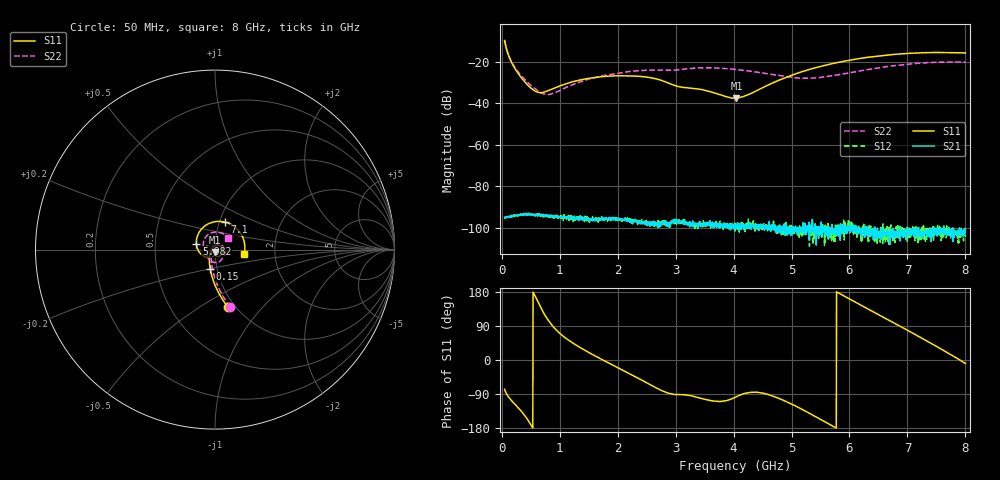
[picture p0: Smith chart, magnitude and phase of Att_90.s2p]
#  HZ  S  DB  R  50.00
! Rohde & Schwarz Vector Network Analyzer
! Rohde-Schwarz,ZNB40-4Port,1311601084101679,3.45
! Created: UTC 4/25/2025, 9:37:07 AM
! freq[Hz]  db:S11  ang:S11  db:S21  ang:S21  db:S12  ang:S12  db:S22  ang:S22
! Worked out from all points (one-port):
!   1750 points, 50 MHz to 8 GHz, reference 50 ohm
!   lowest |S11| = -37.5 dB at 4.05 GHz (marker M1), VSWR 1.03, Z = 49.8 - j1.32 ohm
!   |S11| at or under -10 dB: 52.19 MHz to end of sweep
!   S11 on the Smith chart (normalised r, x): 50 MHz: 0.93, -0.66; 150 MHz: 0.93, -0.20; 5.982 GHz: 0.81, +0.05; 7.1 GHz: 1.06, +0.34; 8 GHz: 1.39, -0.07
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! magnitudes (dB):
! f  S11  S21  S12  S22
! 50 MHz  -9.7  -95.1  -95.2  -9.6
! 150 MHz  -19.0  -94.9  -94.5  -18.9
! 245.5 MHz  -23.9  -94.0  -94.1  -23.4
! 377.3 MHz  -28.9  -93.9  -93.2  -27.8
! 513.6 MHz  -32.8  -93.3  -93.9  -31.5
! 622.7 MHz  -34.6  -93.7  -94.4  -33.9
! 836.4 MHz  -33.5  -94.4  -93.8  -35.6
! 1.377 GHz  -28.6  -95.5  -95.8  -29.4
! 1.995 GHz  -26.7  -95.2  -95.6  -25.5
! 2.423 GHz  -27.1  -97.4  -97.0  -24.1
! 2.7 GHz  -28.4  -99.9  -96.4  -23.9
! 3.05 GHz  -31.9  -96.8  -96.2  -23.8
! 3.505 GHz  -33.7  -98.1  -98.7  -22.8
! 4.027 GHz  -37.5  -98.5  -101.6  -23.6
! 4.05 GHz  -37.5  -98.9  -99.4  -23.7
! 4.282 GHz  -35.4  -99.2  -98.4  -24.4
! 5.036 GHz  -26.1  -100.6  -102.2  -27.6
! 5.35 GHz  -23.3  -99.6  -101.3  -27.8
! 5.982 GHz  -19.3  -100.7  -96.5  -25.3
! 6.677 GHz  -16.6  -105.4  -102.8  -22.1
! 7.1 GHz  -15.7  -102.3  -101.3  -20.8
! 8 GHz  -15.7  -102.0  -104.5  -20.1
